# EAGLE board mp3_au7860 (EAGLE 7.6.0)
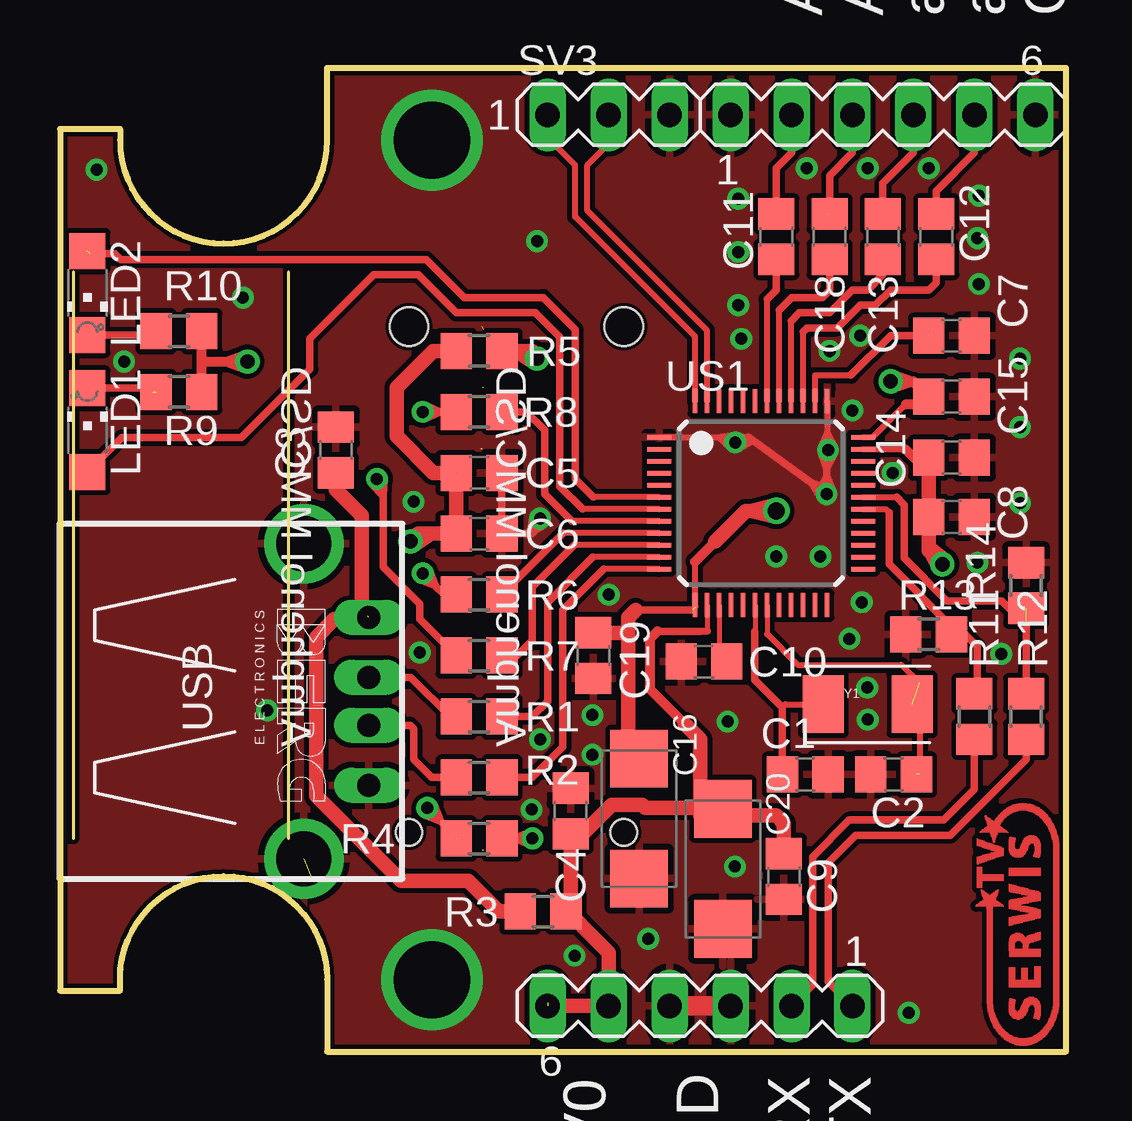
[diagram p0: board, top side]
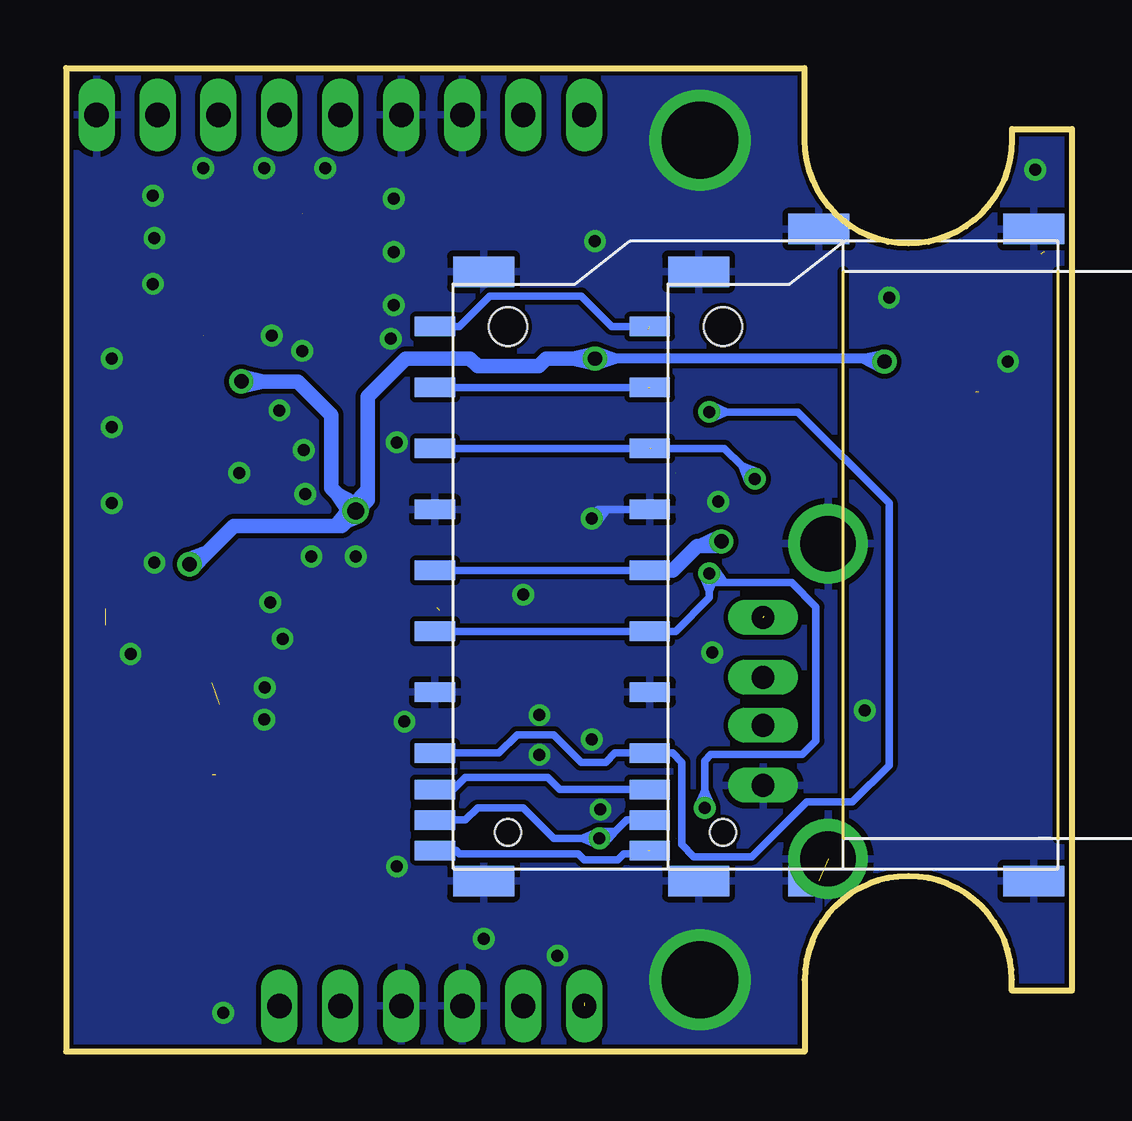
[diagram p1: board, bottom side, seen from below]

Size 41.91 x 41 mm. Coordinates in mm from the lower left corner, seen from the top.
Outline: 2.5,38 2.5,38.46 0,38.46 0,2.54 2.5,2.54 2.5,3
Outline: 2.5,38 arc180 11.13,38
Outline: 2.5,3 arc-180 11.13,3
Outline: 2.5,38 arc180 11.13,38
Outline: 11.13,38 11.13,41 41.91,41 41.91,0 11.13,0 11.13,3
Outline: 2.5,3 arc-180 11.13,3
Copper layers (1*16): Top 0.035mm / dielectric 1.5mm / Bottom 0.035mm
Design rules "default": minimum track width 0mil, minimum drill 22mil, track to track 8mil, track to pad 8mil, pad to pad 8mil, via to via 8mil, smd to smd 8mil, copper to edge 7mil, drill to drill 8mil, minimum pad ring 10mil, minimum via ring 8mil, stop-mask expansion 4mil, vias tented up to drill 23mil, thermal gap 10mil

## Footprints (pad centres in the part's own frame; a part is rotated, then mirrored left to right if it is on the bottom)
C0805 = smd 1.3 x 1.5: 1 -0.95,0; 2 0.95,0
SMC_C = smd 2.4 x 2.4: + -2.5,0; - 2.5,0
CHIPLED_1206 = smd 1.5 x 1.5: A 0,-1.75; C 0,1.75
R0805 = smd 1.3 x 1.5: 1 -0.95,0; 2 0.95,0
MA06-1 = drill 1.016 long: 1 -6.35,0; 2 -3.81,0; 3 -1.27,0; 4 1.27,0; 5 3.81,0; 6 6.35,0
MA03-1 = drill 1.016 long: 1 -2.54,0; 2 0,0; 3 2.54,0
SDCMF-10915W010 = smd 0.813 x 1.676: 1 7.366,13.462; 2 4.826,13.462; 3 2.286,13.462; 4 -0.254,13.462; 5 -2.794,13.462; 6 -5.334,13.462; 7 -7.874,13.462; 8 -9.398,13.462; 9 9.906,13.462; 10 -11.938,13.462; 11 -10.668,13.462 | smd 1.27 x 2.54: 12 12.192,11.43; 13 13.97,-2.54; 14 -13.208,-2.54; 15 -13.208,11.43 | hole 1.6: 9.906,10.414 | hole 1.1: -11.176,10.414
LQFP48-7X7 = smd 1 x 0.2: 1 -4.25,2.75; 2 -4.25,2.25; 3 -4.25,1.75; 4 -4.25,1.25; 5 -4.25,0.75; 6 -4.25,0.25; 7 -4.25,-0.25; 8 -4.25,-0.75; 9 -4.25,-1.25; 10 -4.25,-1.75; 11 -4.25,-2.25; 12 -4.25,-2.75; 25 4.25,-2.75; 26 4.25,-2.25; 27 4.25,-1.75; 28 4.25,-1.25; 29 4.25,-0.75; 30 4.25,-0.25; 31 4.25,0.25; 32 4.25,0.75; 33 4.25,1.25; 34 4.25,1.75; 35 4.25,2.25; 36 4.25,2.75 | smd 0.2 x 1: 13 -2.75,-4.25; 14 -2.25,-4.25; 15 -1.75,-4.25; 16 -1.25,-4.25; 17 -0.75,-4.25; 18 -0.25,-4.25; 19 0.25,-4.25; 20 0.75,-4.25; 21 1.25,-4.25; 22 1.75,-4.25; 23 2.25,-4.25; 24 2.75,-4.25; 37 2.75,4.25; 38 2.25,4.25; 39 1.75,4.25; 40 1.25,4.25; 41 0.75,4.25; 42 0.25,4.25; 43 -0.25,4.25; 44 -0.75,4.25; 45 -1.25,4.25; 46 -1.75,4.25; 47 -2.25,4.25; 48 -2.75,4.25
PN87520-S = drill 0.95 long: 1 -3.5,2.71; 2 -1,2.71; 3 1,2.71; 4 3.5,2.71 | drill 2.3 pad 2.9: S1 -6.57,0; S2 6.57,0
CRYSTAL-TXC-7A = smd 1.7 x 2.4: P$1 1.85,0; P$2 -1.85,0

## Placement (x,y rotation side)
C1  22p  [C0805]  31.05,11.56 180 top
C2  22p  [C0805]  34.73,11.56 0 top
C3  10u  [C0805]  11.49,25.08 90 top
C4  10u  [C0805]  21.27,10.03 90 top
C5  10u  [C0805]  17.46,24.13 0 top
C6  10u  [C0805]  17.46,21.59 0 top
C7  10u  [C0805]  37.15,29.84 0 top
C8  10u  [C0805]  37.15,22.29 0 top
C9  10u  [C0805]  30.16,7.3 270 top
C10  10u  [C0805]  26.83,16.26 180 top
C11  10u  [C0805]  29.84,33.97 270 top
C12  10u  [C0805]  36.51,33.97 270 top
C13  10u  [C0805]  34.29,33.97 270 top
C14  10u  [C0805]  37.15,24.77 0 top
C15  10u  [C0805]  37.15,27.3 0 top
C16  100u/6V niobowy  [SMC_C]  24.13,9.72 270 top
C18  10u  [C0805]  32.07,33.97 270 top
C19  10u  [C0805]  22.23,16.51 270 top
C20  100u/6V niobowy  [SMC_C]  27.62,7.62 270 top
LED1  Zielona  [CHIPLED_1206]  1.14,25.91 0 top
LED2  Czerwona  [CHIPLED_1206]  1.14,31.62 180 top
R1  100  [R0805]  17.46,13.97 0 top
R2  100  [R0805]  17.46,11.43 0 top
R3  1  [R0805]  20.13,5.84 0 top
R4  10k  [R0805]  17.46,8.89 180 top
R5  1  [R0805]  17.46,29.21 0 top
R6  100  [R0805]  17.46,19.05 0 top
R7  100  [R0805]  17.46,16.51 0 top
R8  100  [R0805]  17.46,26.67 0 top
R9  470  [R0805]  4.95,27.5 0 top
R10  470  [R0805]  4.95,30.04 0 top
R11  1  [R0805]  38.1,13.97 90 top
R12  1  [R0805]  40.26,13.97 90 top
R13  nie montowac  [R0805]  36.2,17.4 0 top
R14  nie montowac  [R0805]  40.26,19.43 90 top
SV1  Nie montowac  [MA06-1]  34.29,39.05 0 top
SV2  Nie montowac  [MA06-1]  26.67,1.91 180 top
SV3  [MA03-1]  22.86,39.05 0 top
U$1  Nie montować  [SDCMF-10915W010]  4.13,20.32 90 bottom
U$2  Nie montować  [SDCMF-10915W010]  13.08,20.32 90 bottom
US1  AU7860  [LQFP48-7X7]  29.21,22.86 0 top
USB  Nie montowac  [PN87520-S]  10.16,14.61 270 top
Y1  QSDG12M000-SJK 12MHz www.maritex.com.pl  [CRYSTAL-TXC-7A]  33.66,14.48 0 top

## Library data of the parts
C1-C16 C18-C20 R1-R14 = rcl
LED1 LED2 = led
SV1-SV3 = con-lstb; OC_FARNELL: unknown; OC_NEWARK: unknown
U$1 U$2 = kingfont_sdcmf10915w010_covek
US1 = st-microelectronics
USB = con-berg; OC_FARNELL: unknown; OC_NEWARK: unknown
Y1 = SparkFun-FreqCtrl

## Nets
+3V3: C8.1 C14.1 C15.1 C16.+ C19.1 R5.2 R9.2 R10.2 US1.13 US1.35 US1.36
+5V: C4.1 C9.1 C20.+ R3.2 SV2.5 SV2.6 US1.14
GND: C1.1 C2.1 C3.2 C4.2 C5.2 C6.2 C7.2 C8.2 C9.2 C10.2 C14.2 C15.2 C16.- C19.2 C20.- R13.1 R14.2 SV1.1 SV1.6 SV2.3 SV2.4 SV3.3 U$1.3 U$1.6 U$1.12 U$1.13 U$1.14 U$1.15 U$2.3 U$2.6 U$2.12 U$2.13 U$2.14 U$2.15 US1.1 US1.37 USB.4 USB.S1 USB.S2
N$1: C1.2 US1.18 Y1.P$2
N$2: C2.2 US1.19 Y1.P$1
N$3: R7.1 U$1.2 U$2.2
N$4: C13.2 US1.40
N$5: C12.2 US1.39
N$6: LED2.C R10.1
N$7: LED1.C R9.1
N$8: C7.1 US1.38
N$9: C13.1 SV1.4
N$10: C10.1 US1.15
N$11: C12.1 SV1.5
N$12: R4.1 U$1.11 U$2.11
N$13: R4.2 R6.1 U$1.5 U$2.5
N$14: R8.1 U$1.7 U$2.7
N$15: R11.1 SV2.2
N$16: C5.1 C6.1 R5.1 U$1.4 U$2.4
N$17: C18.2 US1.41
N$18: R11.2 R13.2 US1.30
N$19: R8.2 US1.8
N$20: R7.2 US1.10
N$21: R6.2 US1.9
N$22: R12.1 SV2.1
N$23: C3.1 R3.1 USB.1
N$24: R1.1 USB.2
N$25: R2.1 USB.3
N$26: R12.2 R14.1 US1.31
N$27: R1.2 US1.11
N$28: R2.2 US1.12
N$29: SV3.2 US1.47
N$30: SV3.1 US1.48
N$35: C11.2 US1.42
N$36: C11.1 SV1.2
N$37: C18.1 SV1.3
N$38: LED2.A US1.6
N$39: LED1.A US1.7
N$40: U$1.8 U$2.8
N$41: U$1.9 U$2.9
N$42: U$1.1 U$2.1
N$43: U$1.10 U$2.10

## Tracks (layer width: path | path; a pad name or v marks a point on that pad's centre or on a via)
+3V3  (via drill 0.6, 0.7)  (1 unrouted)
  Top 0.203: 36.2,23.81 36.2,24.13 | 35.88,27.3 C15.1
  Top 0.254: 26.46,20.43 US1.13 26.46,18.52 | US1.35 35.22,25.11 | 35.24,26.99 33.87,25.61 US1.36
  Top 0.305: 36.2,23.81 36.2,22.86 36.2,21.91 C8.1 | 35.88,27.3 35.88,27.62 36.2,27.62 | C15.1 35.88,26.98 35.88,26.99 | 26.35,18.41 24,18.41 | 22.55,17.46 C19.1
  Top 0.406: 26.46,20.43 27.3,21.27 | 35.22,25.11 36.2,24.13 | R9.2 5.9,28.77 | 5.9,28.77 R10.2 | 5.9,28.77 6.91,28.77 | 6.91,28.77 v7.81,28.77 | 35.88,27.62 35.56,27.94 35.51,27.94 | 35.51,27.94 v34.61,27.94 | 35.24,26.99 35.88,26.99 | 23.68,13.02 24.13,12.7 C16.+ | 6.91,28.77 7.71,28.48 v7.81,28.77 | 6.91,28.77 7.71,29.05 v7.81,28.77 | 35.51,27.94 34.71,28.22 v34.61,27.94 | 35.51,27.94 34.71,27.66 v34.61,27.94
  Top 0.61: R5.2 19.03,29.21 | 19.03,29.21 19.68,29.21 v19.88,28.89 | C14.1 36.2,23.81 36.2,21.02 | 36.2,21.02 36.2,20.89 v36.77,20.32 | 23.68,17.46 23.68,18.1 24,18.41 | 23.68,17.46 23.68,13.02 | 22.54,17.46 22.55,17.46 23.68,17.46 | v29.84,22.54 28.8,22.54 | 28.8,22.54 28.57,22.54 27.3,21.27 | 28.8,22.54 29.79,22.3 v29.84,22.54 | 28.8,22.54 29.79,22.78 v29.84,22.54 | 19.03,29.21 19.77,28.73 v19.88,28.89 | 19.03,29.21 19.9,29.09 v19.88,28.89 | 36.2,21.02 36.59,20.23 v36.77,20.32 | 36.2,21.02 36.89,20.48 v36.77,20.32
  Bottom 0.406: 8.7,28.89 8.06,28.89 7.87,28.7 | 8.7,28.89 18.98,28.89 | 18.98,28.89 v19.88,28.89 | 8.7,28.89 7.87,29.06 v7.81,28.77 7.95,28.5 8.7,28.89 | 18.98,28.89 19.77,28.61 v19.88,28.89 | 18.98,28.89 19.77,29.18 v19.88,28.89
  Bottom 0.61: 20.78,28.89 21.91,28.89 22.23,28.57 24.77,28.57 25.08,28.89 27.75,28.89 29.34,27.3 29.34,23.46 | 20.78,28.89 v19.88,28.89 | 33.71,27.94 32.26,27.94 30.86,26.54 30.86,23.5 30.62,23.25 | 33.71,27.94 v34.61,27.94 | v36.77,20.32 36.51,20.32 36.02,20.82 | 36.02,20.82 34.93,21.91 30.68,21.91 | 30.68,21.91 30.42,21.91 29.84,22.48 | 30.62,23.25 29.84,22.48 | 29.34,23.46 29.34,22.99 29.84,22.48 | 30.68,21.91 30.04,22.7 v29.84,22.54 | 30.68,21.91 29.75,22.32 v29.84,22.54 | 30.62,23.25 29.73,22.76 v29.84,22.54 | 30.62,23.25 30.05,22.4 v29.84,22.54 | 29.34,23.46 29.61,22.48 v29.84,22.54 | 29.34,23.46 30.03,22.71 v29.84,22.54 | 20.78,28.89 19.92,29.09 v19.88,28.89 | 20.78,28.89 19.92,28.7 v19.88,28.89 | 36.02,20.82 36.62,20.18 v36.77,20.32 | 36.02,20.82 36.84,20.5 v36.77,20.32 | 33.71,27.94 34.56,27.75 v34.61,27.94 | 33.71,27.94 34.56,28.13 v34.61,27.94
+5V  (1 unrouted)
  Top 0.203: US1.14 26.96,17.54
  Top 0.305: 26.96,17.54 26.67,17.53 24.89,17.53
  Top 0.406: 24.89,17.53 24.57,17.21 24.57,15.11 26.04,13.65 | 26.67,9.84 27.69,9.84 27.69,10.12 | C20.+ 27.69,10.12 | 27.69,10.12 27.69,10.16
  Top 0.61: 20,1.91 SV2.6 SV2.5 22.86,4.13 22.22,4.76 21.27,5.71 | 21.27,5.71 C4.1 21.78,9.08 22.99,10.29 24.26,10.29 24.38,10.16 27.58,10.16 C20.+ | C9.1 30.16,9.53 29.84,9.84 26.67,9.84 26.67,13.02 26.04,13.65 | 20.19,2.16 20.32,2.03 | 21.27,5.71 20.83,6.16 20.83,6.22 R3.2
GND  (via drill 0.5, 3.2)  (1 unrouted)
  Top 0.254: US1.37 31.96,25.83 | 31.96,25.83 31.96,24.66 | US1.1 27.41,25.61 | 27.41,25.61 28.68,25.61 | 31.96,25.83 31.7,25.21 v32,25.08 32.29,25.24 31.96,25.83 | 27.41,25.61 27.91,25.16 v28.13,25.4 28.08,25.72 27.41,25.61
  Top 0.305: C5.2 C6.2 19.6,21.59 | v20,22.23 20,21.91 19.68,21.59 19.6,21.59 | 31.96,24.66 31.96,24.33 | 31.96,24.33 v31.94,23.24 | 28.68,25.61 v31.94,23.24 | 19.6,21.59 20.17,21.98 v20,22.23 | 19.6,21.59 19.7,22.27 v20,22.23 | v31.94,23.24 31.67,23.36 31.95,23.99 32.22,23.36 v31.94,23.24 | v31.94,23.24 31.68,23.09 31.33,23.68 32.01,23.54 v31.94,23.24 | 31.96,24.33 32.27,24.94 v32,25.08 31.72,24.98 31.96,24.33 | 28.88,25.47 28.23,25.68 v28.13,25.4 28.28,25.14 28.88,25.47
  Top 0.813: SV2.3 SV2.4
  Bottom 0.305: U$1.3 19.36,22.61 | 19.36,22.61 19.75,22.61 v20,22.23 | 19.36,22.61 19.76,22.05 v20,22.23 | 19.36,22.61 20.04,22.52 v20,22.23
  other vias: 36.2,36.83 33.66,36.83 31.11,36.83 32.89,17.21 15.5,3 15.5,38 32.07,29.21 33.34,29.84 28.26,35.56 28.26,33.34 34.69,24.13 14.73,22.92 19.88,33.78 24.51,4.7 31.69,20.64 38.23,33.91 2.67,28.77 40.01,28.89 40.01,26.04 40.01,22.86 33.02,26.73 14.99,16.64 29.84,20.64 33.66,13.84 20,13.02 38.29,35.69 28.26,31.11 38.29,32 22.86,19.05 28.12,7.72 39.22,16.57 21.44,4 22.19,14.03 27.81,13.76 7.62,31.43 38.23,20.38 8.64,14.22 1.52,36.77 33.64,15.18 22.19,12.38 19.65,10.09 35.36,1.62 33.4,18.73 28.38,29.72
  pour Bottom: -1.27,41.91 43.18,41.91 43.18,-1.27 -1.27,-1.27
  pour Top: -1.27,41.91 43.18,41.91 43.18,-1.27 -1.27,-1.27
N$1
  Top 0.203: US1.18 28.96,17.53
  Top 0.254: 30.1,14.35 30.23,14.48 Y1.P$2
  Top 0.305: C1.2 30.1,14.35 29.84,14.61 28.96,15.49 28.96,17.53
N$2  (2 unrouted)
  Top 0.203: US1.19 29.46,17.4
  Top 0.254: 29.46,17.4 30.73,16.13 35.05,16.13 35.81,15.37 35.81,11.56
N$3  (via drill 0.5)  (1 unrouted)
  Top 0.305: R7.1 14.99,18.04 14.99,18.67 13.46,20.19 13.46,23.17 | 13.46,23.17 13.46,23.24 13.21,23.5 v13.21,23.88 | 13.46,23.17 13.51,23.86 v13.21,23.88 | 13.46,23.17 12.99,23.67 v13.21,23.88
  Bottom 0.305: v13.21,23.88 13.74,24.41 | 13.74,24.41 14.48,25.15 17.53,25.15 | U$2.2 U$1.2 | 13.74,24.41 13.1,24.16 v13.21,23.88 | 13.74,24.41 13.49,23.77 v13.21,23.88
N$4
  Top 0.254: US1.40 30.46,30.46
  Top 0.305: 30.46,30.46 30.8,30.8 32.07,30.8 33.02,31.75 33.66,31.75 34.29,32.38 C13.2
N$5
  Top 0.254: US1.39 30.96,30.01
  Top 0.305: 30.96,30.01 31.11,30.16 32.38,30.16 33.34,31.11 33.97,31.11 34.61,31.75 36.2,31.75 36.51,32.07 C12.2
N$6
  Top 0.305: LED2.C 4.48,29.87 R10.1
N$7  (1 unrouted)
  Top 0.305: LED1.C 3.52,27.66 3.68,27.5 3.87,27.5
N$8  (1 unrouted)
  Top 0.254: US1.38 31.46,28.19 32.96,28.19
  Top 0.305: 32.96,28.19 34.61,29.84 C7.1
N$9
  Top 0.305: SV1.4 35.56,37.47 34.29,36.2 C13.1
N$10
  Top 0.203: US1.15 27.46,16.51
  Top 0.305: 27.46,16.51 C10.1
N$11
  Top 0.305: SV1.5 38.1,37.47 36.51,35.88 C12.1
N$12  (via drill 0.5)
  Top 0.305: R4.1 18.93,8.89 | 18.93,8.89 v19.68,8.89 | 18.93,8.89 19.56,8.61 v19.68,8.89 | 18.93,8.89 19.56,9.17 v19.68,8.89
  Bottom 0.305: U$1.11 18.54,9.65 19,9.19 | 19,9.19 19.56,8.64 v19.68,8.89 | U$2.11 25.27,9.65 24.77,10.16 22.86,10.16 21.59,8.89 20.43,8.89 | 20.43,8.89 19.94,8.89 19.68,8.64 | 19,9.19 19.46,8.69 v19.68,8.89 | 19,9.19 19.69,9.19 v19.68,8.89 | 20.43,8.89 19.81,9.17 v19.68,8.89 | 20.43,8.89 19.81,8.61 v19.68,8.89
N$13  (via drill 0.5)  (1 unrouted)
  Top 0.305: v15.3,10.16 15.83,9.63 | 15.83,9.63 16.57,8.89 R4.2 | R6.1 16,19.05 15.64,19.41 | 15.64,19.41 v15.11,19.94 | 15.83,9.63 15.58,10.27 v15.3,10.16 | 15.83,9.63 15.19,9.88 v15.3,10.16 | 15.64,19.41 15.39,20.05 v15.11,19.94 | 15.64,19.41 15,19.66 v15.11,19.94
  Bottom 0.305: v15.3,10.16 15.3,10.91 | 15.3,10.91 15.3,12.13 15.05,12.38 11.24,12.38 10.67,12.95 10.67,18.54 11.68,19.56 14.47,19.56 | 14.47,19.56 14.99,19.56 v15.11,19.94 | v15.11,19.94 15.11,19.19 | 15.11,19.19 15.11,18.92 16.51,17.53 U$1.5 U$2.5 | 15.3,10.91 15.03,10.28 v15.3,10.16 | 15.3,10.91 15.58,10.28 v15.3,10.16 | 14.47,19.56 15.15,19.64 v15.11,19.94 | 14.47,19.56 14.87,20.11 v15.11,19.94 | 15.11,19.19 15.39,19.82 v15.11,19.94 | 15.11,19.19 14.84,19.82 v15.11,19.94
N$14  (via drill 0.5)
  Top 0.305: R8.1 15.86,26.67 | 15.86,26.67 v15.11,26.67 | 15.86,26.67 15.23,26.95 v15.11,26.67 | 15.86,26.67 15.23,26.39 v15.11,26.67
  Bottom 0.305: U$2.7 23.88,12.45 23.11,13.21 21.59,13.21 20.45,12.06 19.43,12.06 19.05,12.45 U$1.7 16.64,12.45 16.26,12.06 16.26,8.64 15.75,8.13 13.34,8.13 11.05,10.41 9.14,10.41 7.62,11.94 7.62,22.86 11.43,26.67 14.36,26.67 | v15.11,26.67 14.36,26.67 | 14.36,26.67 14.99,26.39 v15.11,26.67 | 14.36,26.67 14.99,26.95 v15.11,26.67
N$15
  Top 0.305: SV2.2 31.37,2.79 31.37,8.13 32.89,9.65 36.83,9.65 38.1,10.92 R11.1
N$16  (via drill 0.6)  (1 unrouted)
  Top 0.305: C6.1
  Top 0.61: v14.61,21.27 14.92,21.59 15.45,21.59 | 15.45,21.59 C6.1 | R5.1 15.56,29.21 14.03,27.69 14.03,25.65 15.56,24.13 C5.1 | C5.1 C6.1 | 15.45,21.59 14.58,21.47 v14.61,21.27 | 15.45,21.59 14.71,21.11 v14.61,21.27
  Bottom 0.305: U$2.4 U$1.4 17.53,20.07
  Bottom 0.61: v14.61,21.27 14.8,21.27 14.99,21.08 15.48,21.08 | 15.48,21.08 15.62,21.08 16.64,20.07 17.53,20.07 | 15.48,21.08 14.69,21.45 v14.61,21.27 | 15.48,21.08 14.61,21.07 v14.61,21.27
N$17
  Top 0.254: US1.41 29.96,30.91
  Top 0.305: 29.96,30.91 30.48,31.43 31.75,31.43 32.07,31.75 C18.2
N$18
  Top 0.203: 36.96,17.91 36.89,17.65 R13.2
  Top 0.254: US1.30 34.41,22.61 34.54,22.48
  Top 0.305: 34.54,22.48 34.54,20.32 36.96,17.91 | R13.2 37.72,17.4 38.23,16.89 38.23,15.05 R11.2
N$19
  Top 0.254: US1.8 21.32,22.11
  Top 0.305: R8.2 19.43,26.67 20.19,25.91 20.19,23.24 21.32,22.11
N$20
  Top 0.254: US1.10 21.43,21.11
  Top 0.305: 21.43,21.11 19.68,19.37 19.68,17.14 19.05,16.51 R7.2
N$21
  Top 0.254: US1.9 20.98,21.61
  Top 0.305: 18.43,19.07 R6.2 20.98,21.61
N$22
  Top 0.305: SV2.1 32,2.92 32,7.87 33.15,9.02 37.08,9.02 40.26,12.19 R12.1
N$23  (1 unrouted)
  Top 0.61: USB.1 12.8,18.03 11.43,18.03 10.67,17.27 10.67,10.67 14.22,7.11 17.02,7.11 18.29,5.84 R3.1 19.3,6.22 | C3.1 11.49,23.43 12.57,22.35 12.57,18.41 12.83,18.16
N$24
  Top 0.305: R1.1 16.26,13.97 14.62,15.61 USB.2
N$25
  Top 0.305: USB.3 14.59,13.61 14.73,13.46 14.73,12.19 15.49,11.43 R2.1
N$26  (1 unrouted)
  Top 0.254: US1.31 34.87,23.11
  Top 0.305: 34.87,23.11 35.18,22.8 35.18,20.57 36.96,18.8 39.24,18.8 40.26,17.78 R12.2
N$27
  Top 0.254: US1.11 22.2,20.61
  Top 0.305: 22.2,20.61 20.32,18.73 20.32,14.61 19.68,13.97 R1.2
N$28
  Top 0.254: US1.12 22.65,20.11
  Top 0.305: 22.65,20.11 20.95,18.41 20.95,12.7 19.68,11.43 R2.2
N$29
  Top 0.254: US1.47 26.96,30.06 21.97,35.05 21.97,36.96 22.86,37.85 SV3.2
N$30
  Top 0.254: US1.48 26.46,29.8 21.46,34.8 21.46,36.96 20.32,38.1 SV3.1
N$35
  Top 0.254: US1.42 29.46,31.36
  Top 0.305: 29.46,31.36 29.84,31.75 C11.2
N$36
  Top 0.305: SV1.2 30.48,37.47 29.84,36.83 C11.1
N$37  (1 unrouted)
  Top 0.305: SV1.3 33.02,37.47 32.07,36.51 C18.1 | 32.38,35.24 C18.1
N$38  (1 unrouted)
  Top 0.254: US1.6 22.23,23.11
  Top 0.305: 22.23,23.11 21.46,23.88 21.46,30.1 20.13,31.43 16.84,31.43 15.25,33.02 2.54,33.02 2.29,33.27 1.27,33.27
N$39
  Top 0.254: US1.7 21.78,22.61
  Top 0.305: LED1.A 2.58,25.59 7.56,25.59 10.41,28.45 10.41,29.72 13.08,32.38 14.92,32.38 16.51,30.8 19.81,30.8 20.83,29.78 20.83,23.56 21.78,22.61
N$40
  Bottom 0.305: U$2.8 25.78,10.92 25.27,11.43 21.84,11.43 21.34,10.92 U$1.8
N$41  (1 unrouted)
  Bottom 0.305: U$2.9 25.53,30.23 24.26,31.5 20.45,31.5 19.18,30.23 17.78,30.23 17.65,30.1
N$42  (1 unrouted)
  Bottom 0.305: U$2.1 17.65,27.69
N$43  (1 unrouted)
  Bottom 0.305: U$2.10 25.65,8.38 25.53,8.26 20.57,8.26 20.32,8 18.92,8 18.67,8.26 17.78,8.26 17.65,8.38 17.65,8.26
(copper drawn outside any net)
  shapes: Top area x895

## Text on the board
tPlace: AUX left channel in - connect to GND | AUX right channel in - connect to GND | audio left channel output | audio right channel output | GND | 5V0 | GND | RX | TX
tStop: MP3 | v.1.3

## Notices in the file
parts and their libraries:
SparkFun-FreqCtrl: Licensing: CC v3.0 Share-Alike You are welcome to use this library for commercial purposes.
